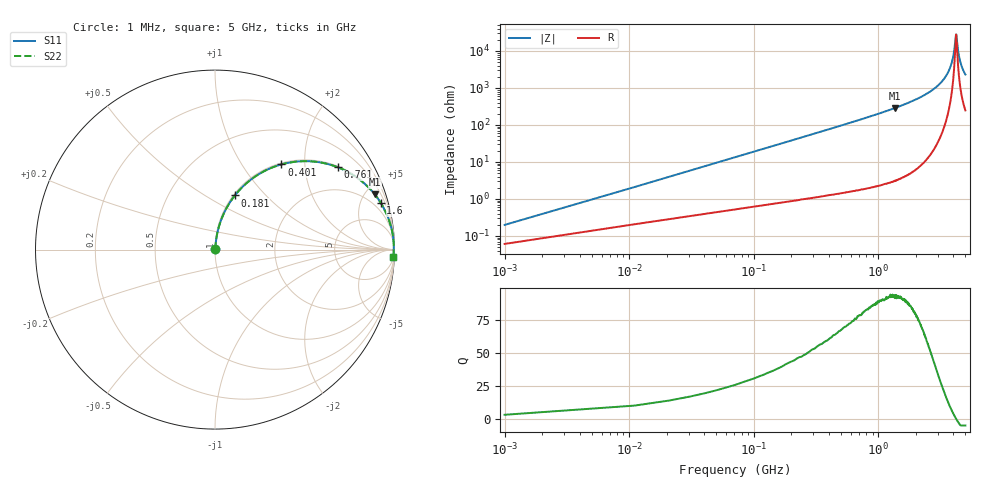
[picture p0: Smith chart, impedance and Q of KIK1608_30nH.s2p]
!version-2
!date-01.2022
!Series
# MHz S RI R 50
!Freq ReS11 ImS11 ReS21 ImS21 ReS12 ImS12 ReS22 ImS22
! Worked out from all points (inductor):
!   501 points, 1 MHz to 5 GHz, reference 50 ohm
!   read as one part in series: L = 30 nH near 21 MHz
!   highest Q = 93.6 at 1.37 GHz (marker M1), where L = 33.6 nH
!   self-resonance near 4.21 GHz
!   S11 on the Smith chart (normalised r, x): 1 MHz: 1.00, +0.00; 181 MHz: 1.02, +0.68; 401 MHz: 1.03, +1.53; 761 MHz: 1.04, +2.97; 1.6 GHz: 1.08, +7.05; 5 GHz: 6, -46
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1  0.000618 0.00188  0.9994 -0.00188  0.9994 -0.00188  0.000618 0.00188
31  0.00678 0.0578  0.9932 -0.0578  0.9932 -0.0578  0.00678 0.0578
51  0.0134 0.0944  0.9866 -0.0944  0.9866 -0.0944  0.0134 0.0944
101  0.0405 0.1816  0.9595 -0.1816  0.9595 -0.1816  0.0405 0.1816
181  0.1104 0.3016  0.8896 -0.3016  0.8896 -0.3016  0.1104 0.3016
401  0.3699 0.4746  0.6301 -0.4746  0.6301 -0.4746  0.3699 0.4746
761  0.6853 0.4583  0.3147 -0.4583  0.3147 -0.4583  0.6853 0.4583
841  0.7292 0.4385  0.2708 -0.4385  0.2708 -0.4385  0.7292 0.4385
1370  0.8905 0.307  0.1095 -0.307  0.1095 -0.307  0.8905 0.307
1600  0.9231 0.2609  0.0769 -0.2609  0.0769 -0.2609  0.9231 0.2609
1670  0.9308 0.2483  0.0692 -0.2483  0.0692 -0.2483  0.9308 0.2483
2510  0.9795 0.1332  0.0205 -0.1332  0.0205 -0.1332  0.9795 0.1332
3340  0.9938 0.0585  0.00619 -0.0585  0.00619 -0.0585  0.9938 0.0585
3660  0.9957 0.0354  0.00425 -0.0354  0.00425 -0.0354  0.9957 0.0354
3890  0.9964 0.0201  0.00362 -0.0201  0.00362 -0.0201  0.9964 0.0201
4050  0.9965 0.00998  0.00348 -0.00998  0.00348 -0.00998  0.9965 0.00998
4170  0.9965 0.00268  0.00352 -0.00268  0.00352 -0.00268  0.9965 0.00268
4200  0.9964 0.000891  0.00355 -0.000891  0.00355 -0.000891  0.9964 0.000891
4230  0.9964 -0.000886  0.00359 0.000886  0.00359 0.000886  0.9964 -0.000886
4390  0.9961 -0.0101  0.00388 0.0101  0.00388 0.0101  0.9961 -0.0101
4560  0.9956 -0.0196  0.00439 0.0196  0.00439 0.0196  0.9956 -0.0196
5000  0.9936 -0.0426  0.00645 0.0426  0.00645 0.0426  0.9936 -0.0426
